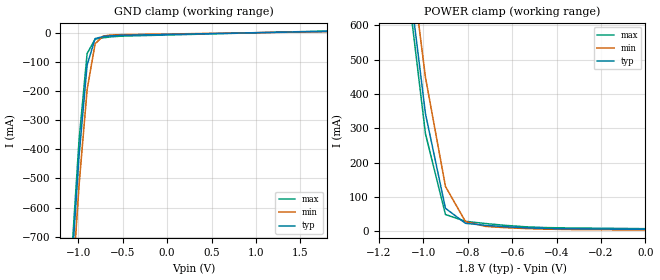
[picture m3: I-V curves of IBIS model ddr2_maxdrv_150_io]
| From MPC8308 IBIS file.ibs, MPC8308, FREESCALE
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[Model]   ddr2_maxdrv_150_io   |
Model_type   Input
Vinl = 0.87
Vinh = 0.93
| variable   typ   min   max
C_comp   1.17p   1.10p   1.23p
[Model Spec]
| subparameter   typ   min   max
S_overshoot_high  3.300   3.135   3.465
S_overshoot_low   -200.00m  -100.00m  -300.00m
D_overshoot_high  4.000   4.000   4.000
D_overshoot_low   -1.000   -1.000   -1.000
D_overshoot_time  1.000n   1.000n   1.000n
| variable   typ   min   max
[Temperature Range]   55.0   110.0   0.0
| variable   typ   min   max
[Pullup Reference]   1.800V   1.710V   1.890V
| variable   typ   min   max
[Pulldown Reference]   0.000V   0.000V   0.000V
| variable   typ   min   max
[POWER_Clamp_Reference]   1.800V   1.710V   1.890V
| variable   typ   min   max
[GND_Clamp_Reference]   0.000V   0.000V   0.000V
[GND_clamp]
|Voltage   I(typ)   I(min)   I(max)
-1.89V    -5.299A    -5.32A     -5.304A
-1.08V    -839.8mA   -930.8mA   -793.6mA
-990mV    -420.8mA   -521mA     -365.6mA
-900mV    -110.7mA   -194.8mA   -71.07mA
-810mV    -19.66mA   -37.49mA   -21.41mA
-720mV    -12.5mA    -10.88mA   -16.82mA
-630mV    -10.13mA   -7.452mA   -13.68mA
1.8V      5.099mA    3.684mA    6.383mA
[POWER_clamp]
|Voltage   I(typ)   I(min)   I(max)
-1.71V    4.948A     4.961A     4.962A
-1.08V    817.3mA    912.2mA    770.9mA
-990mV    342.7mA    448.9mA    284.2mA
-900mV    66.48mA    130.3mA    48.37mA
-810mV    22.76mA    27.72mA    28.58mA
-720mV    16.77mA    13.74mA    22.06mA
-450mV    7.634mA    5.725mA    10.19mA
-2.22fV   5.099mA    3.394mA    7.007mA
